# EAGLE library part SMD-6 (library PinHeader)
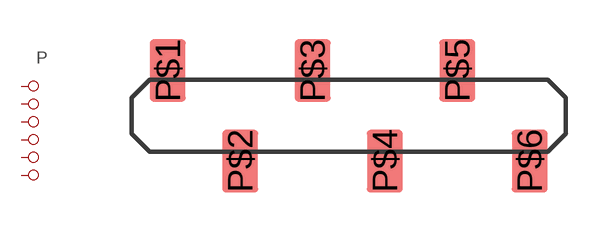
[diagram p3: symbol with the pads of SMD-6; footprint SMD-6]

Designator prefix P

## SMD-6  [SMD-6]
P$1  1  pas
P$2  2  pas
P$3  3  pas
P$4  4  pas
P$5  5  pas
P$6  6  pas

## Footprint SMD-6 (pad centres in mm)
smd 1.27 x 2.2: P$1 -6.35,1.587; P$2 -3.81,-1.587; P$3 -1.27,1.587; P$4 1.27,-1.587; P$5 3.81,1.587; P$6 6.35,-1.587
